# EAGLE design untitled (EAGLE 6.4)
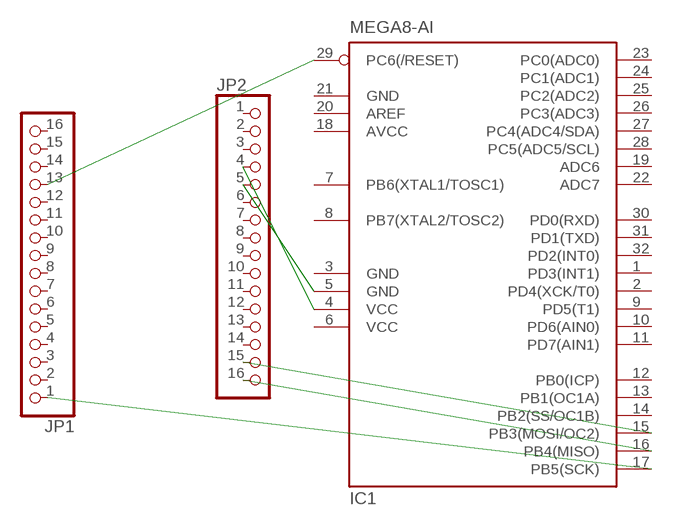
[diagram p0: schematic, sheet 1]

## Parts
IC1  MEGA8-AI  [TQFP32-08]
JP1  PINHD-1X16  [1X16]
JP2  PINHD-1X16  [1X16]

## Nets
N$4: IC1.4(VCC) JP2.4
N$5: IC1.5(GND) JP2.5
N$15: IC1.15(PB3(MOSI/OC2)) JP2.15
N$16: IC1.16(PB4(MISO)) JP2.16
N$17: IC1.17(PB5(SCK)) JP1.1
N$29: IC1.29(PC6(/RESET)) JP1.13
Unconnected: IC1.1(PD3(INT1)) IC1.2(PD4(XCK/T0)) IC1.7(PB6(XTAL1/TOSC1)) IC1.8(PB7(XTAL2/TOSC2)) IC1.9(PD5(T1)) IC1.10(PD6(AIN0)) IC1.11(PD7(AIN1)) IC1.12(PB0(ICP)) IC1.13(PB1(OC1A)) IC1.14(PB2(SS/OC1B)) IC1.19(ADC6) IC1.20(AREF) IC1.22(ADC7) IC1.23(PC0(ADC0)) IC1.24(PC1(ADC1)) IC1.25(PC2(ADC2)) IC1.26(PC3(ADC3)) IC1.27(PC4(ADC4/SDA)) IC1.28(PC5(ADC5/SCL)) IC1.30(PD0(RXD)) IC1.31(PD1(TXD)) IC1.32(PD2(INT0)) JP1.2 JP1.3 JP1.4 JP1.5 JP1.6 JP1.7 JP1.8 JP1.9 JP1.10 JP1.11 JP1.12 JP1.14 JP1.15 JP1.16 JP2.1 JP2.2 JP2.3 JP2.6 JP2.7 JP2.8 JP2.9 JP2.10 JP2.11 JP2.12 JP2.13 JP2.14

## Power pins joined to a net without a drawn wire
AVCC: IC1.18(AVCC)
GND: IC1.3(GND) IC1.21(GND)
VCC: IC1.6(VCC)

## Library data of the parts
IC1 = atmel:MEGA8: MICROCONTROLLER 8 Kbytes FLASH, 1 kbytes SRAM, 512 bytes EEPROM, USART, 6-channel 10 bit ADC, 2-channel 8 bit ADC Pin compatible with Atmega48, ATMega88, ATMega168 Source: avr.lbr; MPN: ATMEGA8-16AU; OC_FARNELL: 9171371; OC_NEWARK: 73M8863
JP1 JP2 = pinhead:PINHD-1X16: PIN HEADER

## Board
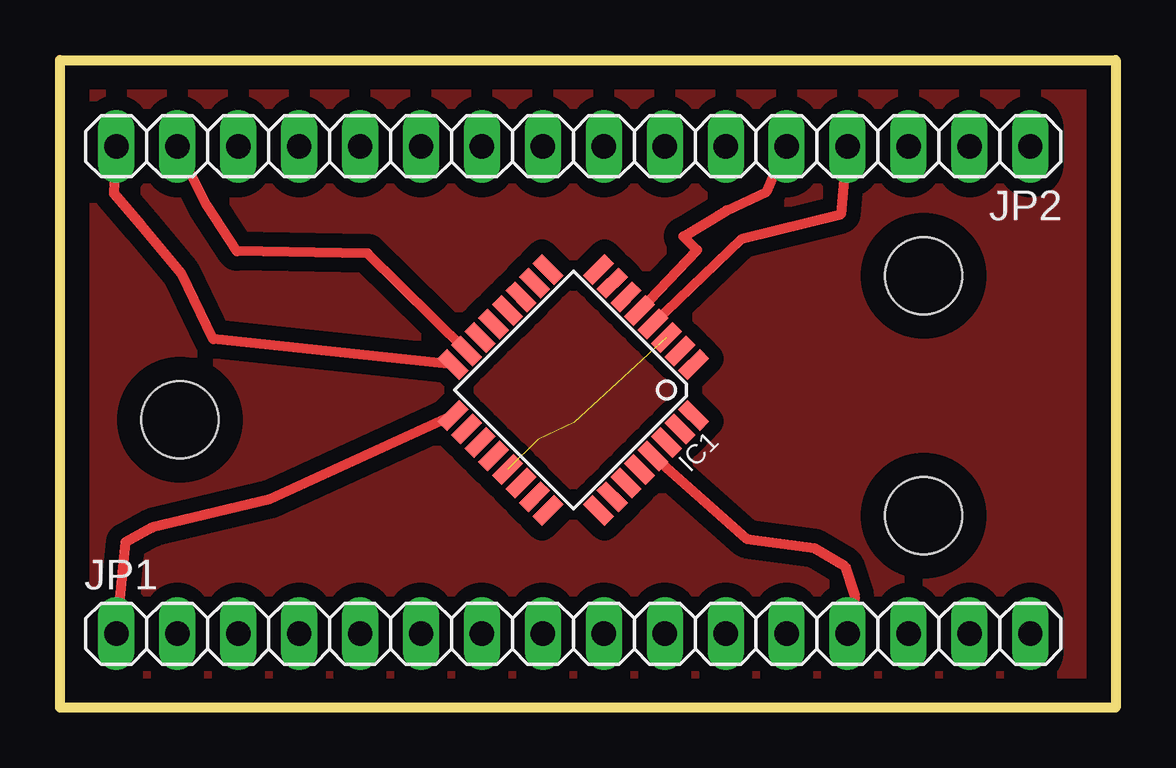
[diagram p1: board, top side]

Size 44 x 27 mm. Coordinates in mm from the lower left corner, seen from the top.
Outline: 0,0 0,27 44,27 44,0 0,0
Copper layers (1*16): Top 0.035mm / dielectric 1.5mm / Bottom 0.035mm
Design rules "default": minimum track width 10mil, minimum drill 24mil, track to track 8mil, track to pad 8mil, pad to pad 8mil, via to via 8mil, smd to smd 8mil, copper to edge 40mil, drill to drill 8mil, minimum pad ring 10mil, minimum via ring 8mil, stop-mask expansion 4mil, vias tented up to drill 0mil, thermal gap 10mil
Holes 3.2 mm at 5,12 36,18 36,8

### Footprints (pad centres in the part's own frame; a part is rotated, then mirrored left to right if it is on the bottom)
TQFP32-08 = smd 1.27 x 0.559: 1 -4.293,2.8; 2 -4.293,2; 3 -4.293,1.2; 4 -4.293,0.4; 5 -4.293,-0.4; 6 -4.293,-1.2; 7 -4.293,-2; 8 -4.293,-2.8; 17 4.293,-2.8; 18 4.293,-2; 19 4.293,-1.2; 20 4.293,-0.4; 21 4.293,0.4; 22 4.293,1.2; 23 4.293,2; 24 4.293,2.8 | smd 0.559 x 1.27: 9 -2.8,-4.293; 10 -2,-4.293; 11 -1.2,-4.293; 12 -0.4,-4.293; 13 0.4,-4.293; 14 1.2,-4.293; 15 2,-4.293; 16 2.8,-4.293; 25 2.8,4.293; 26 2,4.293; 27 1.2,4.293; 28 0.4,4.293; 29 -0.4,4.293; 30 -1.2,4.293; 31 -2,4.293; 32 -2.8,4.293
1X16 = drill 1.016 long: 1 -19.05,0; 2 -16.51,0; 3 -13.97,0; 4 -11.43,0; 5 -8.89,0; 6 -6.35,0; 7 -3.81,0; 8 -1.27,0; 9 1.27,0; 10 3.81,0; 11 6.35,0; 12 8.89,0; 13 11.43,0; 14 13.97,0; 15 16.51,0; 16 19.05,0

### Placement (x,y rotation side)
IC1  21.4,13.24 225 top
JP1  21.4,3.08 0 top
JP2  21.4,23.4 180 top

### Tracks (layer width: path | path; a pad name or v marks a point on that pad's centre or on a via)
GND  (3 unrouted)
N$1
  pour Top (isolate 0.61): 1,26 43,26 43,1 1,1
N$4
  Top 0.406: IC1.4 28.43,19.54 32.57,20.58 JP2.4
N$5
  Top 0.406: IC1.5 26.55,19.07 25.99,19.64 27.77,20.72 29.47,21.52 JP2.5
N$15
  Top 0.406: IC1.15 12.83,18.93 7.38,19.03 6.11,20.95 JP2.15
N$16
  Top 0.406: IC1.16 6.39,15.36 5.07,18.09 3.38,20.11 2.25,21.43 JP2.16
N$17
  Top 0.406: IC1.17 8.74,8.68 3.85,7.5 2.72,6.89 JP1.1
N$29
  Top 0.406: IC1.29 28.62,7.03 31.44,6.66 32.71,5.9 33.13,4.63 JP1.13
